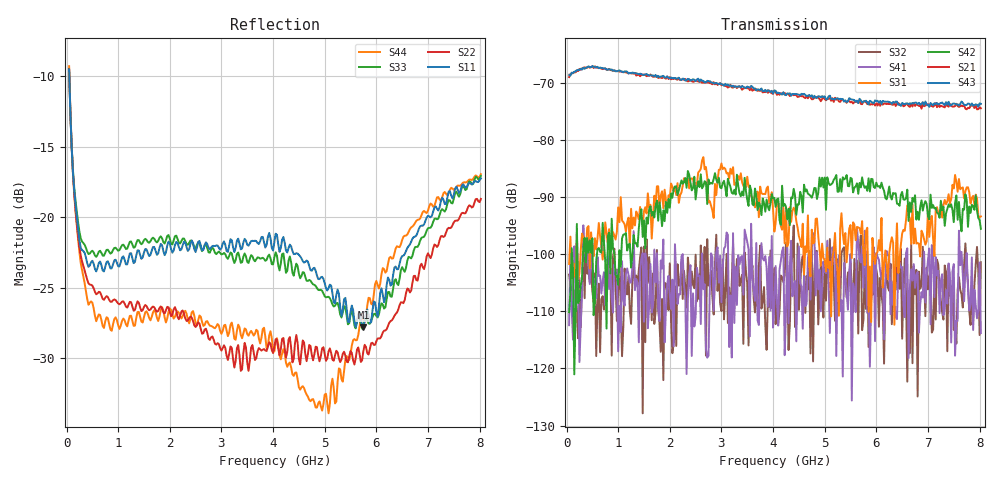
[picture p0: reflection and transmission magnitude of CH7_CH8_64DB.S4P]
!Agilent Technologies,E5071C,MY46316741,A.11.02
!Date: Mon Jun 01 10:27:10 2026
!Data & Calibration Information:
!1:CH7 INPUT 2:CH7 OUTPUT 3:CH8 INPUT 4:CH8 OUTPUT
!Freq	S11:SOLT4(ON)	S12:SOLT4(ON)	S13:SOLT4(ON)	S14:SOLT4(ON)
!	S21:SOLT4(ON)	S22:SOLT4(ON)	S23:SOLT4(ON)	S24:SOLT4(ON)
!	S31:SOLT4(ON)	S32:SOLT4(ON)	S33:SOLT4(ON)	S34:SOLT4(ON)
!	S41:SOLT4(ON)	S42:SOLT4(ON)	S43:SOLT4(ON)	S44:SOLT4(ON)
!PortZ  Port1:50+j0  Port2:50+j0  Port3:50+j0  Port4:50+j0
!Above PortZ is port z conversion or system Z0 setting when saving the data.
!When reading, reference impedance value at option line is always used.
# Hz S dB R 50
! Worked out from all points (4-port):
!   320 points, 50 MHz to 8.025 GHz, reference 50 ohm
!   strongest paths, dB at 50 MHz, 2.05 GHz, 4.05 GHz, 6.05 GHz, 8.025 GHz:
!     S43: -68.6, -69.2, -71.4, -73.5, -73.7
!     S21: -69.0, -69.3, -71.6, -73.4, -74.5
!     S42: -110.2, -90.1, -91.7, -88.1, -95.6
!     S31: -101.7, -88.2, -94.5, -97.6, -93.4
!     S41: -112.4, -104.5, -102.1, -101.0, -113.8
!     S32: -103.6, -117.3, -112.3, -112.7, -101.4
!   lowest |S11| = -27.8 dB at 5.75 GHz (marker M1), VSWR 1.08, Z = 47.2 - j2.77 ohm
!   |S11| at or under -10 dB: 53.89 MHz to end of sweep
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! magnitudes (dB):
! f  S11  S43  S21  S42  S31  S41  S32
! 50 MHz  -9.5  -68.6  -69.0  -110.2  -101.7  -112.4  -103.6
! 250 MHz  -21.6  -67.8  -67.6  -108.0  -103.3  -118.9  -104.1
! 725 MHz  -23.8  -67.5  -67.5  -97.9  -98.1  -103.2  -109.7
! 3.825 GHz  -21.8  -71.4  -71.6  -91.1  -89.5  -101.1  -105.8
! 5.075 GHz  -25.0  -72.4  -72.8  -87.5  -102.5  -104.6  -104.2
! 5.75 GHz  -27.8  -73.3  -73.3  -87.8  -99.8  -105.9  -111.5
! 8.025 GHz  -17.2  -73.7  -74.5  -95.6  -93.4  -113.8  -101.4
